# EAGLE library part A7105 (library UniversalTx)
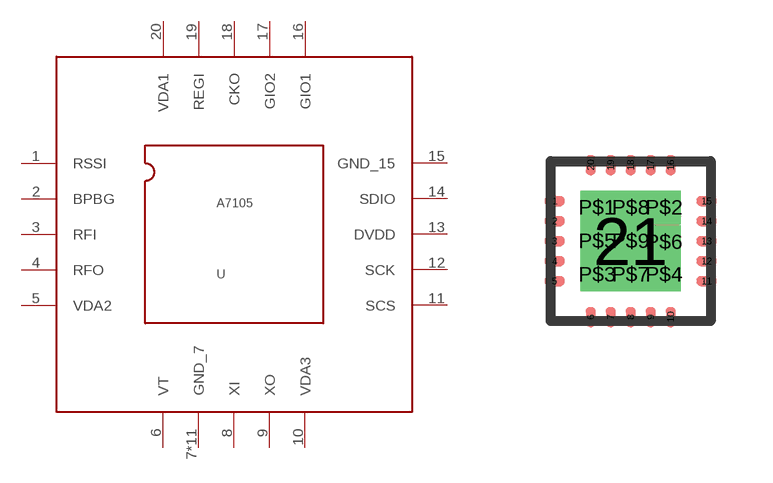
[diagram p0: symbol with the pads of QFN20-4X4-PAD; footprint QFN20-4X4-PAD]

Designator prefix -

## A7105  [QFN20-4X4-PAD]
1  RSSI
2  BPBG
3  RFI
4  RFO
5  VDA2
6  VT
7  GND_7
8  XI
9  XO
10  VDA3
11  SCS
12  SCK
13  DVDD
14  SDIO
15  GND_15
16  GIO1
17  GIO2
18  CKO
19  REGI
20  VDA1
21  GND_7
P$1  GND_7
P$2  GND_7
P$3  GND_7
P$4  GND_7
P$5  GND_7
P$6  GND_7
P$7  GND_7
P$8  GND_7
P$9  GND_7

## Footprint QFN20-4X4-PAD (pad centres in mm)
QFN20 4mm x 4mm package, with matt tin plating from Nordic Semiconductor.
smd 0.5 x 0.25: 1 -1.9,1; 2 -1.9,0.5; 3 -1.9,0; 4 -1.9,-0.5; 5 -1.9,-1; 11 1.9,-1; 12 1.9,-0.5; 13 1.9,0; 14 1.9,0.5; 15 1.9,1
smd 0.25 x 0.5: 6 -1,-1.9; 7 -0.5,-1.9; 8 0,-1.9; 9 0.5,-1.9; 10 1,-1.9; 16 1,1.9; 17 0.5,1.9; 18 0,1.9; 19 -0.5,1.9; 20 -1,1.9
smd 2.4 x 2.4: 21 0,0
drill 0.33 pad 0.686 square: P$1 -0.838,0.838; P$2 0.838,0.838; P$3 -0.838,-0.838; P$4 0.838,-0.838; P$5 -0.838,0; P$6 0.838,-0.025; P$7 0,-0.838; P$8 0,0.838; P$9 0,0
